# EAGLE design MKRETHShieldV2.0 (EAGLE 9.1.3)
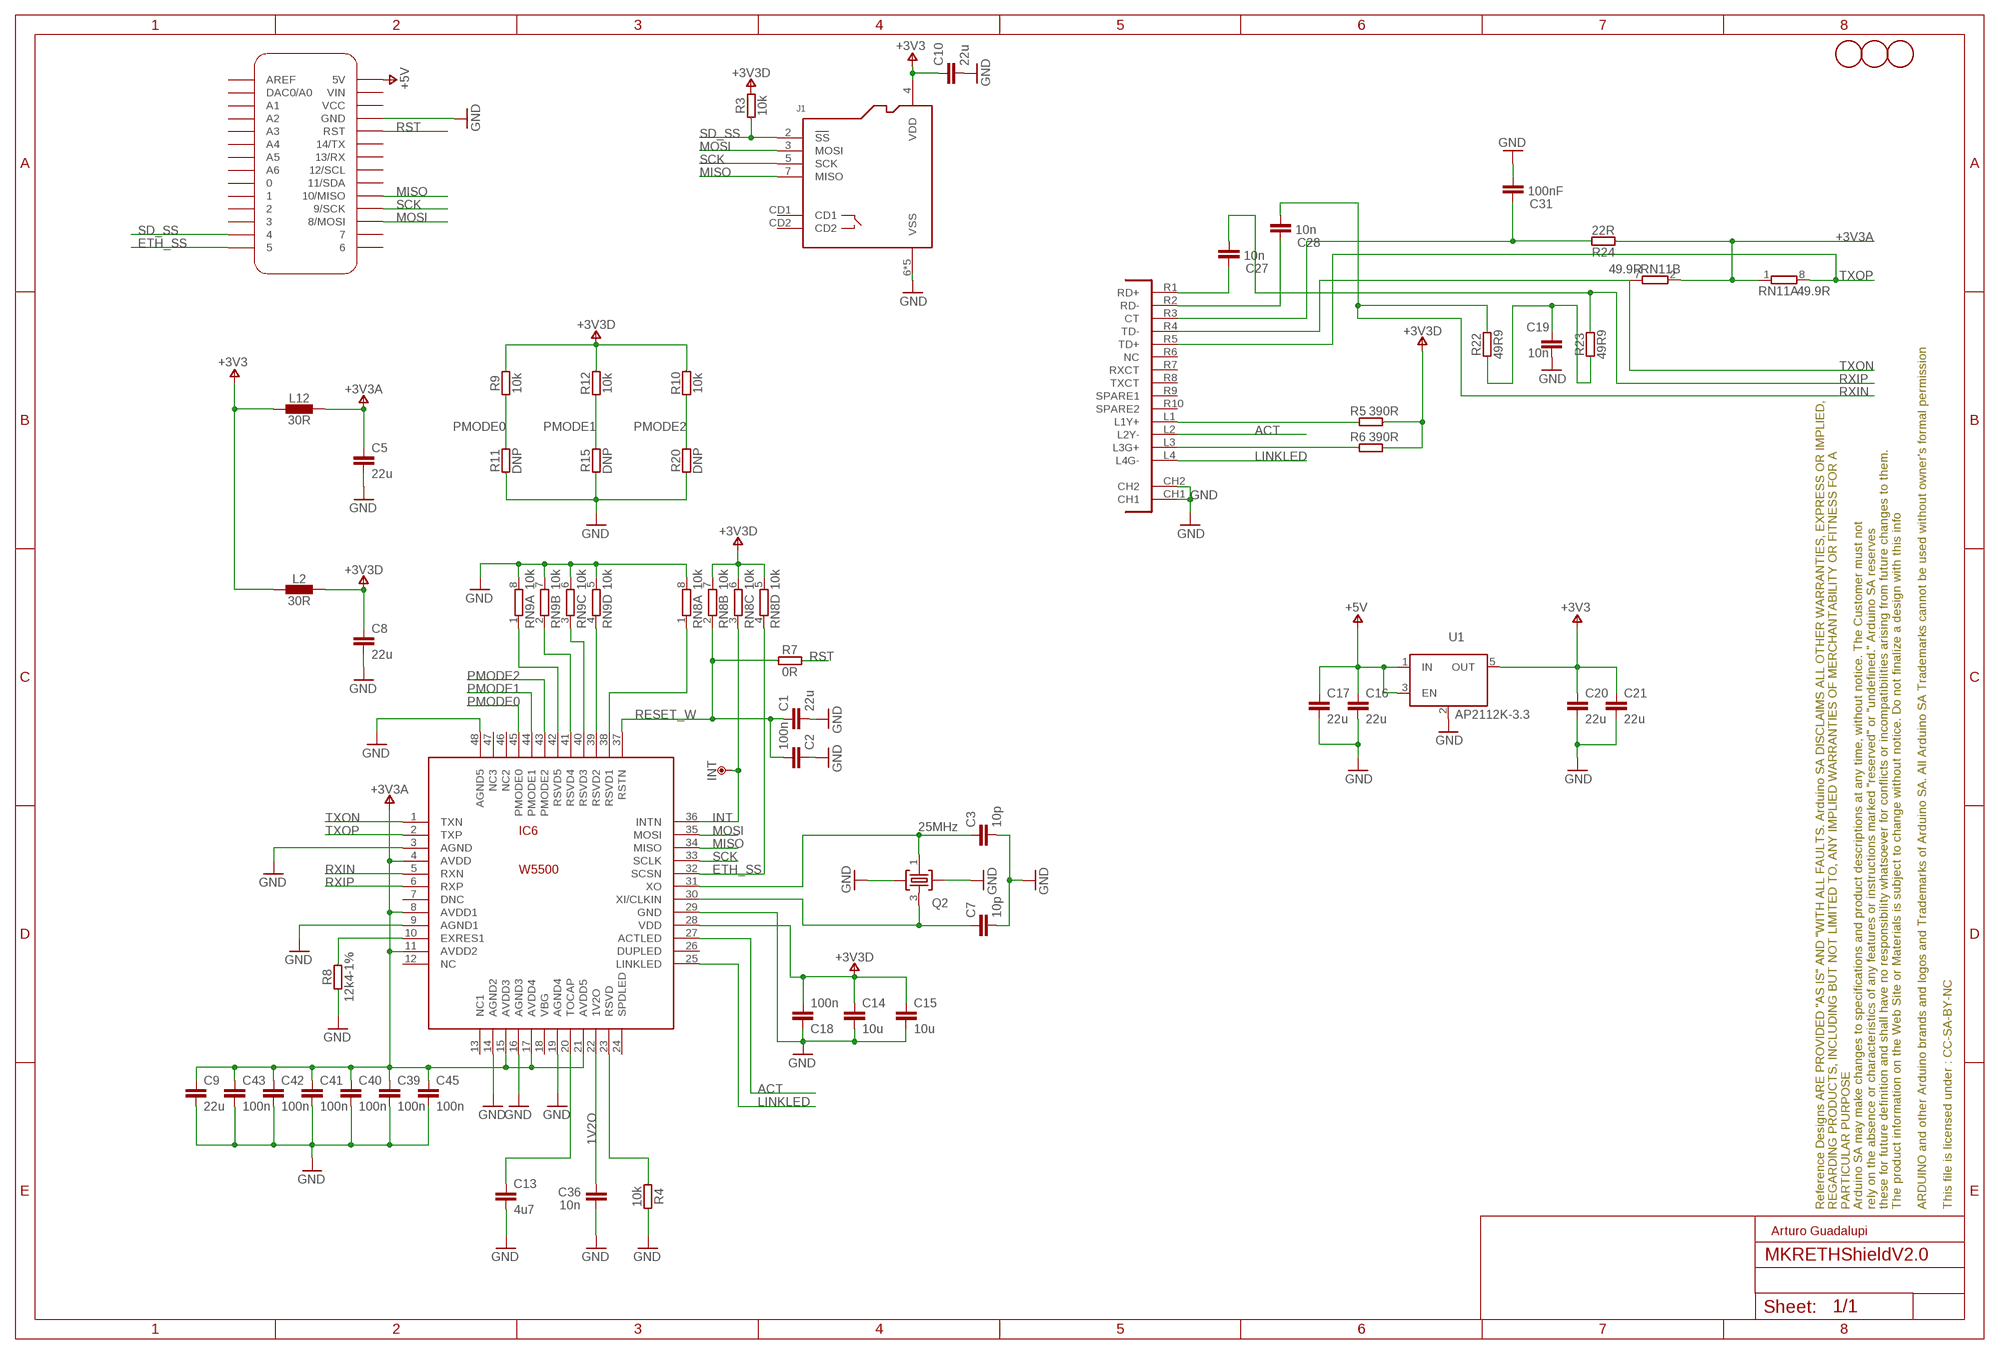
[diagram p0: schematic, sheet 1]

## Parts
C1  22u  C-22U-0805  [0805-R2013X50N]
C2  100n  C-100NF-0402  [0402-1005X55N]
C3  10p  C-10PF-0402  [0402-1005X55N]
C5  22u  C-22U-0805  [0805-R2013X50N]
C7  10p  C-10PF-0402  [0402-1005X55N]
C8  22u  C-22U-0805  [0805-R2013X50N]
C9  22u  C-22U-0805  [0805-R2013X50N]
C10  22u  C-22U-0805  [0805-R2013X50N]
C13  4u7  C-4.7UF-0603  [0603-1608X90N]
C14  10u  C-10UF-0603  [0603-1608X90N]
C15  10u  C-10UF-0603  [0603-1608X90N]
C16  22u  C-22U-0805  [0805-R2013X50N]
C17  22u  C-22U-0805  [0805-R2013X50N]
C18  100n  C-100NF-0402  [0402-1005X55N]
C19  10n  C-10NF-0402  [0402-1005X55N]
C20  22u  C-22U-0805  [0805-R2013X50N]
C21  22u  C-22U-0805  [0805-R2013X50N]
C27  10n  C-10NF-0402  [0402-1005X55N]
C28  10n  C-10NF-0402  [0402-1005X55N]
C31  100nF  C-100NF-0402  [0402-1005X55N]
C36  10n  C-10NF-0402  [0402-1005X55N]
C39  100n  C-100NF-0402  [0402-1005X55N]
C40  100n  C-100NF-0402  [0402-1005X55N]
C41  100n  C-100NF-0402  [0402-1005X55N]
C42  100n  C-100NF-0402  [0402-1005X55N]
C43  100n  C-100NF-0402  [0402-1005X55N]
C45  100n  C-100NF-0402  [0402-1005X55N]
FRAME1  DNP  A3-FRAME-STANDARD  [FRAME]
IC6  W5500  [TQFP48-7X7]
INT  DNP  TPTP-1.27MM  [TP-1.27MM]
J1  -  SD_AMPHENOL-SPI  [AMPHENOL_114-00841-68]
L2  30R  FERRITE-30R0805  [0805-R2013X50N]
L12  30R  FERRITE-30R0805  [0805-R2013X50N]
MKR1  DNP  MKRBOARD-DNP-DIM  [MKRBOARD-DIM]
Q2  25MHz  25MHZ  [CRYSTAL3.2X2.5]
R3  10k  R-10K-0402  [0402-1005X55N]
R4  10k  R-10K-0402  [0402-1005X55N]
R5  390R  R-390R-0402  [0402-1005X55N]
R6  390R  R-390R-0402  [0402-1005X55N]
R7  0R  R-0R-0402  [0402-1005X55N]
R8  12k4-1%  R12K4-1%-0402  [0402-1005X55N]
R9  10k  R-10K-0402  [0402-1005X55N]
R10  10k  R-10K-0402  [0402-1005X55N]
R11  DNP  R-DNP-0402  [0402-1005X55N]
R12  10k  R-10K-0402  [0402-1005X55N]
R15  DNP  R-DNP-0402  [0402-1005X55N]
R20  DNP  R-DNP-0402  [0402-1005X55N]
R22  49R9  R-49R9-0402  [0402-1005X55N]
R23  49R9  R-49R9-0402  [0402-1005X55N]
R24  22R  R-22R-0402  [0402-1005X55N]
RN8  10k  4R-N-10KCAY16  [CAY16]
RN9  10k  4R-N-10KCAY16  [CAY16]
RN11  49.9R  4R-N-49.9RCAY16  [CAY16]
U1  AP2112K-3.3  [SOT25]
U$1  DNP  FIDUCIAL-1.5MM  [FD-1-1.5]
U$2  DNP  FIDUCIAL-1.5MM  [FD-1-1.5]
U$3  DNP  FIDUCIAL-1.5MM  [FD-1-1.5]
UC1  -  ETH-CON-RB1-125BHQ1A  [POE-RJ45]

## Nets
1V2O: C36.2 IC6.22(1V2O)
+3V3 [power]: C10.1 C20.1 C21.1 J1.4(VDD) L2.1 L12.1 U1.5(OUT)
+3V3A [power]: C5.1 C9.1 C39.1 C40.1 C41.1 C42.1 C43.1 C45.1 IC6.4(AVDD) IC6.8(AVDD1) IC6.11(AVDD2) IC6.15(AVDD3) IC6.17(AVDD4) IC6.21(AVDD5) L12.2 R24.1 RN11.1 RN11.2
+3V3D: C8.1 C14.1 C15.1 C18.2 IC6.28(VDD) L2.2 R3.2 R5.2 R6.2 R9.2 R10.2 R12.2 RN8.5 RN8.6 RN8.7
+5V [power]: C16.1 C17.1 MKR1.5V U1.1(IN) U1.3(EN)
ACT: IC6.27(ACTLED) UC1.L2(L2Y-)
ETH_SS: IC6.32(SCSN) MKR1.5 RN8.4
GND [power]: C1.2 C2.1 C3.2 C5.2 C7.2 C8.2 C9.2 C10.2 C13.2 C14.2 C15.2 C16.2 C17.2 C18.1 C19.1 C20.2 C21.2 C31.1 C36.1 C39.2 C40.2 C41.2 C42.2 C43.2 C45.2 IC6.3(AGND) IC6.9(AGND1) IC6.14(AGND2) IC6.16(AGND3) IC6.19(AGND4) IC6.29(GND) IC6.48(AGND5) J1.6(VSS) J1.SH1(VSS) J1.SH2(VSS) J1.SH3(VSS) J1.SH4(VSS) MKR1.GND Q2.2 Q2.4 R4.1 R8.1 R11.1 R15.1 R20.1 RN8.8 RN9.5 RN9.6 RN9.7 RN9.8 U1.2(GND/ADJ) UC1.CH1 UC1.CH2
INT: IC6.36(INTN) INT.X RN8.3
LINKLED: IC6.25(LINKLED) UC1.L4(L4G-)
MISO: IC6.34(MISO) J1.7(MISO) MKR1.10(10/MISO)
MOSI: IC6.35(MOSI) J1.3(MOSI) MKR1.8(8/MOSI)
N$9: C3.1 IC6.31(XO) Q2.1
N$13: IC6.39(RSVD2) RN9.4
N$22: R6.1 UC1.L3(L3G+)
N$24: IC6.23(RSVD) R4.2
N$25: R5.1 UC1.L1(L1Y+)
N$26: C19.2 R22.1 R23.1
N$27: C27.2 UC1.R1(RD+)
N$28: C28.2 UC1.R2(RD-)
N$31: IC6.40(RSVD3) RN9.3
N$35: IC6.41(RSVD4) RN9.2
N$36 [power]: C31.2 R24.2 UC1.R3(CT)
N$37: IC6.42(RSVD5) RN9.1
N$38: C13.1 IC6.20(TOCAP)
N$39: IC6.38(RSVD1) RN8.1
N$40: IC6.10(EXRES1) R8.2
OSC2E2: C7.1 IC6.30(XI/CLKIN) Q2.3
PMODE0: IC6.45(PMODE0) R9.1 R11.2
PMODE1: IC6.44(PMODE1) R12.1 R15.2
PMODE2: IC6.43(PMODE2) R10.1 R20.2
RESET_W: C1.1 C2.2 IC6.37(RSTN) R7.1 RN8.2
RST: MKR1.RST R7.2
RXIN: C28.1 IC6.5(RXN) R22.2
RXIP: C27.1 IC6.6(RXP) R23.2
SCK: IC6.33(SCLK) J1.5(SCK) MKR1.9(9/SCK)
SD_SS: J1.2(SS) MKR1.4 R3.1
TXON: IC6.1(TXN) RN11.7 UC1.R4(TD-)
TXOP: IC6.2(TXP) RN11.8 UC1.R5(TD+)
Unconnected: IC6.7(DNC) IC6.13(NC1) IC6.18(VBG) IC6.24(SPDLED) IC6.46(NC2) IC6.47(NC3) J1.CD1 J1.CD2 MKR1.0 MKR1.1 MKR1.2 MKR1.3 MKR1.6 MKR1.7 MKR1.11(11/SDA) MKR1.12(12/SCL) MKR1.13(13/RX) MKR1.14(14/TX) MKR1.A0(DAC0/A0) MKR1.A1 MKR1.A2 MKR1.A3 MKR1.A4 MKR1.A5 MKR1.A6 MKR1.AREF MKR1.VCC MKR1.VIN RN11.3 RN11.4 RN11.5 RN11.6 UC1.R6(NC) UC1.R7(RXCT) UC1.R8(TXCT) UC1.R9(SPARE1) UC1.R10(SPARE2)

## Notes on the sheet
- Arturo Guadalupi

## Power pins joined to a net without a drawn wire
DUPLED: IC6.26(DUPLED)
NC: IC6.12(NC)

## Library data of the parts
C1 C5 C8-C10 C16 C17 C20 C21 = Arduino-rcl:C: SMD Capacitor; CODE-ARDUINO: 2233; DATASHEET: https://media.digikey.com/pdf/Data%20Sheets/Samsung%20PDFs/CL21A226MQCLQNC_character.pdf; DISTRIBUTOR-LINK: https://www.digikey.com/product-detail/en/samsung-electro-mechanics-america-inc/CL21A226MQCLQNC/1276-2412-1-ND/3890498; DISTRIBUTOR-PN: 1276-2412-1-ND; MANUFACTURER: Samsung; MANUFACTURER-PN: CL21A226MQCLQNC
C2 C18 C31 C39-C43 C45 = Arduino-rcl:C: SMD Capacitor; CODE-ARDUINO: 0132; DATASHEET: http://www.tdk.com/pdf/TDKMLCCCapRange.pdf; DISTRIBUTOR-LINK: http://www.digikey.com/product-detail/en/tdk-corporation/C1005X5R1H104K050BB/445-5942-1-ND/2443982; DISTRIBUTOR-PN: 445-5942-1-ND; MANUFACTURER: TDK; MANUFACTURER-PN: C1005X5R1H104K050BB
C3 C7 = Arduino-rcl:C: SMD Capacitor; CODE-ARDUINO: 3382; DATASHEET: http://search.murata.co.jp/Ceramy/image/img/A01X/partnumbering_e_01.pdf; DISTRIBUTOR-LINK: https://www.digikey.com/product-detail/en/murata-electronics-north-america/GRM1555C1H100FA01D/490-6186-1-ND/3845386; DISTRIBUTOR-PN: 490-6186-1-ND; MANUFACTURER: Murata; MANUFACTURER-PN: GRM1555C1H100FA01D
C13 = Arduino-rcl:C: SMD Capacitor; CODE-ARDUINO: 0458; DATASHEET: http://www.murata.com/~/media/webrenewal/support/library/catalog/products/capacitor/mlcc/c02e.pdf; DISTRIBUTOR-LINK: http://www.digikey.com/product-search/en?keywords=490-7203-1-ND; DISTRIBUTOR-PN: 490-7203-1-ND; MANUFACTURER: Murata; MANUFACTURER-PN: GRM188R61E475KE11D
C14 C15 = Arduino-rcl:C: SMD Capacitor; CODE-ARDUINO: 2213; DATASHEET: http://www.murata.com/~/media/webrenewal/support/library/catalog/products/capacitor/mlcc/c02e.pdf; DISTRIBUTOR-LINK: http://www.digikey.com/product-search/en?keywords=490-10728-1-ND; DISTRIBUTOR-PN: 490-10728-1-ND; MANUFACTURER: Murata; MANUFACTURER-PN: GRM188R61C106KAALD
C19 C27 C28 C36 = Arduino-rcl:C: SMD Capacitor; CODE-ARDUINO: 0165; DATASHEET: http://search.murata.co.jp/Ceramy/image/img/A01X/partnumbering_e_01.pdf; DISTRIBUTOR-LINK: http://www.digikey.com/product-detail/en/murata-electronics-north-america/GRM155R71H103KA88J/490-6351-1-ND/3845548; DISTRIBUTOR-PN: 490-6351-1-ND; MANUFACTURER: Murata; MANUFACTURER-PN: GRM155R71H103KA88J
FRAME1 = Arduino-utility:A3-FRAME: Schematic frame; CODE-ARDUINO: DNP; DATASHEET: DNP; DISTRIBUTOR-LINK: DNP; DISTRIBUTOR-PN: DNP; MANUFACTURER: DNP; MANUFACTURER-PN: DNP
IC6 = Arduino-ICs:W5500: W5500 Hardwired TCP/IP Ethernet controller; CODE-ARDUINO: 0982; DATASHEET: http://wizwiki.net/wiki/lib/exe/fetch.php?media=products:w5500:w5500_ds_v106e_141230.pdf; DISTRIBUTOR-LINK: https://www.digikey.com/product-detail/en/wiznet/W5500/1278-1021-ND/4425702; DISTRIBUTOR-PN: 1278-1021-ND; MANUFACTURER: WizNet; MANUFACTURER-PN: W5500
INT = Arduino-utility:TP: Testpoint; DATASHEET: DNP; DISTRIBUTOR-LINK: DNP; DISTRIBUTOR-PN: DNP; MANUFACTURER: DNP; MANUFACTURER-PN: DNP
J1 = Arduino-connectors:SD_AMPHENOL-SPI: Micro SD connector; CODE-ARDUINO: 0046; DATASHEET: https://www.amphenolcanada.com/ProductSearch/drawings/AC/1140084168.pdf; DISTRIBUTOR-LINK: http://www.digikey.com/product-detail/en/amphenol-commercial-products/114-00841-68/114-00841-68-1-ND/2187101; DISTRIBUTOR-PN: 114-00841-68-1-ND; MANUFACTURER: Amphenol; MANUFACTURER-PN: 114-00841-68
L2 L12 = Arduino-rcl:FERRITE: SMD ferrite; CODE-ARDUINO: 0001; DATASHEET: https://media.digikey.com/pdf/Data%20Sheets/Samsung%20PDFs/Chip_Inductor_Catalog_2014.pdf; DISTRIBUTOR-LINK: https://www.digikey.com/products/en?keywords=CIB21P300NE; DISTRIBUTOR-PN: CIB21P300NE-ND; MANUFACTURER: Samsung; MANUFACTURER-PN: CIB21P300NE
MKR1 = Arduino-utility:MKRBOARD: MKR board footprint; DATASHEET: DNP; DISTRIBUTOR-LINK: DNP; DISTRIBUTOR-PN: DNP; MANUFACTURER: DNP; MANUFACTURER-PN: DNP
Q2 = Arduino-crystals:25MHZ: 25Mhz - K7 12pF - SMD; CODE-ARDUINO: 2359; DATASHEET: https://abracon.com/Resonators/ABM8G.pdf; DISTRIBUTOR-LINK: https://www.digikey.com/product-detail/en/abracon-llc/ABM8G-25.000MHZ-B4Y-T/535-10297-1-ND/2218110; DISTRIBUTOR-PN: 535-10297-1-ND; MANUFACTURER: Abracon LLC; MANUFACTURER-PN: ABM8G-25.000MHZ-B4Y-T
R3 R4 R9 R10 R12 = Arduino-rcl:R: SMD Resistor; CODE-ARDUINO: 0136; DATASHEET: www.yageo.com.tw/exep/pages/download/literatures/PYu-R_INT-thick_7.pdf; DISTRIBUTOR-LINK: http://www.digikey.com/product-detail/en/yageo/RC0402FR-0710KL/311-10.0KLRCT-ND/729470; DISTRIBUTOR-PN: 311-10.0KLRCT-ND; MANUFACTURER: Yageo; MANUFACTURER-PN: RC0402FR-0710KL; _RESTRICTIONS: NO
R5 R6 = Arduino-rcl:R: SMD Resistor; CODE-ARDUINO: 2195; DATASHEET: www.yageo.com.tw/exep/pages/download/literatures/PYu-R_INT-thick_7.pdf; DISTRIBUTOR-LINK: https://www.digikey.com/product-detail/en/yageo/RC0402FR-07390RL/311-390LRCT-ND/2827929; DISTRIBUTOR-PN: 311-390LRCT-ND; MANUFACTURER: Yageo; MANUFACTURER-PN: RC0402FR-07390RL; _RESTRICTIONS: NO
R7 = Arduino-rcl:R: SMD Resistor; CODE-ARDUINO: 0039; DATASHEET: www.yageo.com.tw/exep/pages/download/literatures/PYu-R_INT-thick_7.pdf; DISTRIBUTOR-LINK: http://www.digikey.com/product-detail/en/yageo/RC0402FR-070RL/311-0.0LRCT-ND/2827888; DISTRIBUTOR-PN: 311-0.0LRCT-ND; MANUFACTURER: Yageo; MANUFACTURER-PN: RC0402FR-070RL; _RESTRICTIONS: NO
R8 = Arduino-rcl:R: SMD Resistor; CODE-ARDUINO: 2297; DATASHEET: http://www.yageo.com/NewPortal/yageodocoutput?fileName=/pdf/R-Chip/PYu-RC_Group_51_RoHS_L_4.pdf; DISTRIBUTOR-LINK: https://www.digikey.com/product-detail/en/yageo/RC0402FR-0712K4L/311-12.4KLRCT-ND/2827940; DISTRIBUTOR-PN: 311-12.4KLRCT-ND; MANUFACTURER: Yageo; MANUFACTURER-PN: RC0402FR-0712K4L; _RESTRICTIONS: 1% only
R11 R15 R20 = Arduino-rcl:R: SMD Resistor; CODE-ARDUINO: DNP; DATASHEET: DNP; DISTRIBUTOR-LINK: DNP; DISTRIBUTOR-PN: DNP; MANUFACTURER: DNP; MANUFACTURER-PN: DNP; _RESTRICTIONS: NO
R22 R23 = Arduino-rcl:R: SMD Resistor; CODE-ARDUINO: A5282; DATASHEET: www.yageo.com.tw/exep/pages/download/literatures/PYu-R_INT-thick_7.pdf; DISTRIBUTOR-LINK: https://www.digikey.com/product-detail/en/yageo/RC0402FR-0749R9L/311-49.9LRCT-ND/729568; DISTRIBUTOR-PN: 311-49.9LRCT-ND; MANUFACTURER: Yageo; MANUFACTURER-PN: RC0402FR-0749R9L; _RESTRICTIONS: 1% ONLY
R24 = Arduino-rcl:R: SMD Resistor; CODE-ARDUINO: 0468; DATASHEET: www.yageo.com.tw/exep/pages/download/literatures/PYu-R_INT-thick_7.pdf; DISTRIBUTOR-LINK: http://www.digikey.com/products/en?keywords=311-22.0LRCT-ND; DISTRIBUTOR-PN: 311-22.0LRCT-ND; MANUFACTURER: Yageo; MANUFACTURER-PN: RC0402FR-0722RL; _RESTRICTIONS: NO
RN8 RN9 = Arduino-rcl:4R-N: Array Chip Resistor Source: RS Component / Phycomp; CODE-ARDUINO: 0016; DATASHEET: http://www.bourns.com/docs/Product-Datasheets/CATCAY.pdf; DISTRIBUTOR-LINK: https://www.digikey.com/products/en?keywords=CAY16-103J4LFTR-ND; DISTRIBUTOR-PN: CAY16-103J4LFTR-ND; MANUFACTURER: Bourns Inc.; MANUFACTURER-PN: CAY16-103J4LF
RN11 = Arduino-rcl:4R-N: Array Chip Resistor Source: RS Component / Phycomp; CODE-ARDUINO: 2298; DATASHEET: http://www.bourns.com/docs/Product-Datasheets/CATCAY.pdf; DISTRIBUTOR-LINK: https://www.digikey.com/product-detail/en/bourns-inc/CAY16-49R9F4LF/CAY16-49R9F4LFCT-ND/3437972; DISTRIBUTOR-PN: CAY16-49R9F4LFCT-ND; MANUFACTURER: Bourns Inc.; MANUFACTURER-PN: CAY16-49R9F4LF
U1 = Arduino-ICs:AP2112K-3.3: IC REG LINEAR 3.3V 600mA SOT25; CODE-ARDUINO: 2199; DATASHEET: https://www.diodes.com/assets/Datasheets/AP2112.pdf; DISTRIBUTOR-LINK: https://www.digikey.com/product-detail/en/diodes-incorporated/AP2112K-3.3TRG1/AP2112K-3.3TRG1DITR-ND/4470746; DISTRIBUTOR-PN: AP2112K-3.3TRG1DITR-ND; MANUFACTURER: Diodes Inc; MANUFACTURER-PN: AP2112K-3.3TRG1
U$1-U$3 = Arduino-utility:FIDUCIAL: Fiducial mount; CODE-ARDUINO: DNP; DATASHEET: DNP; DISTRIBUTOR-LINK: DNP; DISTRIBUTOR-PN: DNP; MANUFACTURER: DNP; MANUFACTURER-PN: DNP
UC1 = Arduino-connectors:ETH-CON-RB1-125BHQ1A: RJ45 connector; CODE-ARDUINO: 2300; DATASHEET: https://www2.mouser.com/datasheet/2/443/RB1-125BAG1A(111-00)-1211926.pdf; DISTRIBUTOR-LINK: https://www2.mouser.com/ProductDetail/WIZnet/RB1-125BAG1A?qs=K8aI8m0%252bj2HL3CgJHC4yWQ%3D%3D; DISTRIBUTOR-PN: 950-RB1-125BAG1A; MANUFACTURER: Wiznet; MANUFACTURER-PN: RB1-125BAG1A

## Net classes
1 power: width 0.254 mm, drill 0.3 mm, clearance 0.203 mm
2 gnd: width 0.254 mm, drill 0.3 mm, clearance 0.254 mm

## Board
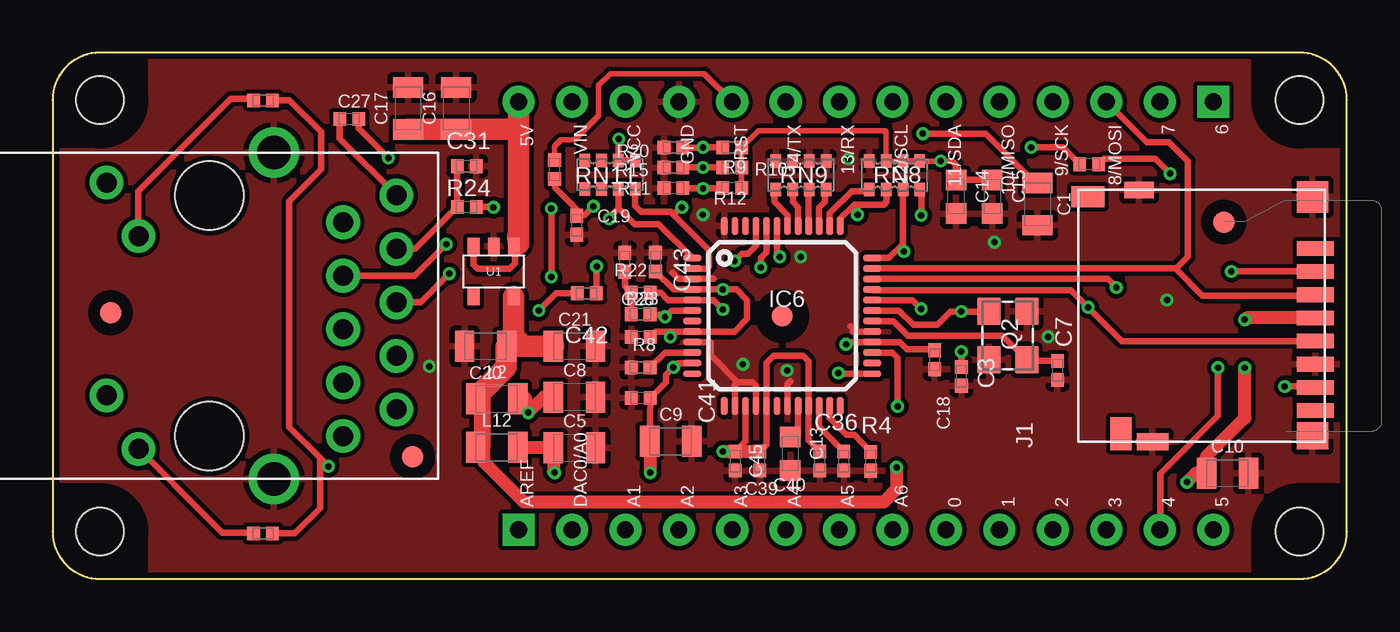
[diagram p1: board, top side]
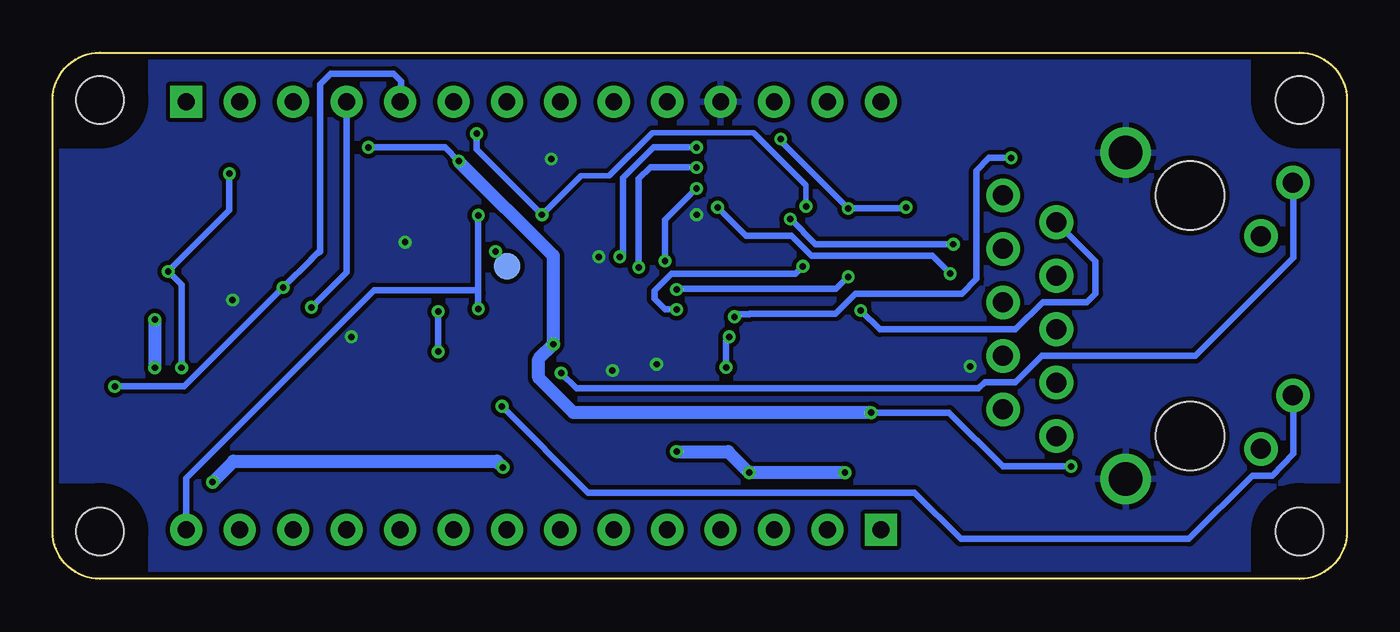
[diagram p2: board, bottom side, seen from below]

Size 61.5 x 25 mm. Coordinates in mm from the lower left corner, seen from the top.
Copper layers (1*16): Top 0.035mm / dielectric 1.5mm / Bottom 0.035mm
Design rules "SeeedStudio_2layers *": minimum track width 6mil, minimum drill 12mil, track to track 7mil, track to pad 6mil, pad to pad 6mil, via to via 6mil, smd to smd 0mil, copper to edge 10mil, drill to drill 10mil, minimum pad ring 10mil, minimum via ring 6mil, stop-mask expansion 2mil, vias tented up to drill 100mil, thermal gap 10mil

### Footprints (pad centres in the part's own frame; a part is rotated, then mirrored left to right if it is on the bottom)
0805-R2013X50N = smd 0.95 x 1.45: 1 -1,0; 2 1,0
0402-1005X55N = smd 0.62 x 0.62: 1 -0.45,0; 2 0.45,0
0603-1608X90N = smd 0.95 x 1: 1 -0.8,0; 2 0.8,0
TQFP48-7X7 = smd 0.85 x 0.32: 1 -4.275,2.75; 2 -4.275,2.25; 3 -4.275,1.75; 4 -4.275,1.25; 5 -4.275,0.75; 6 -4.275,0.25; 7 -4.275,-0.25; 8 -4.275,-0.75; 9 -4.275,-1.25; 10 -4.275,-1.75; 11 -4.275,-2.25; 12 -4.275,-2.75; 25 4.275,-2.75; 26 4.275,-2.25; 27 4.275,-1.75; 28 4.275,-1.25; 29 4.275,-0.75; 30 4.275,-0.25; 31 4.275,0.25; 32 4.275,0.75; 33 4.275,1.25; 34 4.275,1.75; 35 4.275,2.25; 36 4.275,2.75 | smd 0.32 x 0.85: 13 -2.75,-4.275; 14 -2.25,-4.275; 15 -1.75,-4.275; 16 -1.25,-4.275; 17 -0.75,-4.275; 18 -0.25,-4.275; 19 0.25,-4.275; 20 0.75,-4.275; 21 1.25,-4.275; 22 1.75,-4.275; 23 2.25,-4.275; 24 2.75,-4.275; 37 2.75,4.275; 38 2.25,4.275; 39 1.75,4.275; 40 1.25,4.275; 41 0.75,4.275; 42 0.25,4.275; 43 -0.25,4.275; 44 -0.75,4.275; 45 -1.25,4.275; 46 -1.75,4.275; 47 -2.25,4.275; 48 -2.75,4.275 | smd 1 x 1: P$1 0,0
TP-1.27MM = smd 1.27 x 1.27 bottom: X 0,0
AMPHENOL_114-00841-68 = smd 0.7 x 1.75: 1 3.2,-5.888; 2 2.1,-5.888; 3 1,-5.888; 4 -0.1,-5.888; 5 -1.2,-5.888; 6 -2.3,-5.888; 7 -3.4,-5.888; 8 -4.5,-5.888 | smd 1 x 1.55: CD1 5.65,4.912 | smd 1.55 x 1: CD2 -5.602,3.337 | smd 1.3 x 1.5: SH1 -5.7,-5.76 | smd 1.5 x 1.5: SH2 5.65,-5.76 | smd 0.8 x 1.4: SH3 5.975,2.487 | smd 0.8 x 1.5: SH4 -5.975,1.837
MKRBOARD-DIM = drill 0.8 pad 1.524: 0 42.455,2.34; 1 44.995,2.34; 2 47.535,2.34; 3 50.075,2.34; 4 52.615,2.34; 5 55.155,2.34; 5V 22.135,22.66; 7 52.615,22.66; 8 50.075,22.66; 9 47.535,22.66; 10 44.995,22.66; 11 42.455,22.66; 12 39.915,22.66; 13 37.375,22.66; 14 34.835,22.66; A0 24.675,2.34; A1 27.215,2.34; A2 29.755,2.34; A3 32.295,2.34; A4 34.835,2.34; A5 37.375,2.34; A6 39.915,2.34; GND 29.755,22.66; RST 32.295,22.66; VCC 27.215,22.66; VIN 24.675,22.66 | drill 0.8 pad 1.524 square: 6 55.155,22.66; AREF 22.135,2.34 | hole 2.25: 59.25,2.25; 59.25,22.75; 2.25,2.25; 2.25,22.75
CRYSTAL3.2X2.5 = smd 1.3 x 1.1: 1 -1.15,-0.9; 2 1.15,-0.9; 3 1.15,0.9; 4 -1.15,0.9
CAY16 = smd 0.5 x 0.65: 1 -1.2,-0.675; 2 -0.4,-0.675; 3 0.4,-0.675; 4 1.2,-0.675; 5 1.2,0.675; 6 0.4,0.675; 7 -0.4,0.675; 8 -1.2,0.675
SOT25 = smd 0.55 x 0.8: 1 0.95,1.2; 2 0,1.2; 3 -0.95,1.2; 4 -0.95,-1.2; 5 0.95,-1.2
FD-1-1.5 = smd 1.016 x 1.016: P$1 0,0
POE-RJ45 = drill 1.6: CH1 13.94,7.75; CH2 13.94,-7.75 | drill 0.95 pad 1.6: L1 7.51,-6.325; L2 5.99,-3.785; L3 7.51,3.785; L4 5.99,6.325; R1 19.77,5.715; R2 17.23,4.445; R3 19.77,3.175; R4 17.23,1.905; R5 19.77,0.635; R6 17.23,-0.635; R7 19.77,-1.905; R8 17.23,-3.175; R9 19.77,-4.445; R10 17.23,-5.715 | hole 3.25: 10.89,5.715; 10.89,-5.715

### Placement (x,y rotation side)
C1  46.8,17.8 270 top
C2  24.9,16.8 90 top
C3  43.18,9.62 270 top
C5  24.8,6.22 0 top
C7  47.75,9.91 270 top
C8  24.8,8.64 0 top
C9  29.37,6.54 0 top
C10  55.82,5.02 0 top
C13  35.05,5.95 270 top
C14  42.93,18.15 270 top
C15  44.65,18.15 270 top
C16  19.18,22.35 90 top
C17  16.89,22.35 90 top
C18  41.91,10.41 90 top
C19  27.19,15.04 270 top
C20  20.57,11.05 180 top
C21  24.8,11.05 0 top
C27  14.1,21.84 180 top
C28  25.38,13.57 180 top
C31  19.68,19.6 180 top
C36  37.59,5.6 90 top
C39  33.6,5.6 270 top
C40  36.45,5.6 270 top
C41  27.95,8.6 180 top
C42  27.95,11.5 180 top
C43  28.65,15.05 90 top
C45  32.43,5.6 270 top
FRAME1  not placed on the board
IC6  34.67,12.5 0 top
INT  39.9,14.85 0 top
J1  54.1,12.5 90 top
L2  21.1,8.55 0 top
L12  21.1,6.25 0 top
MKR1  0,0 0 top
Q2  45.39,11.56 270 top
R3  49.25,19.7 180 top
R4  38.87,5.59 90 top
R5  10,2.16 0 top
R6  10,22.73 0 top
R7  23.85,19.45 90 top
R8  27.94,10.04 0 top
R9  32.29,18.57 0 top
R10  32.29,20.49 0 top
R11  29.5,18.57 0 top
R12  32.29,19.54 0 top
R15  29.5,19.54 0 top
R20  29.5,20.49 0 top
R22  27.95,13.59 0 top
R23  27.94,12.57 0 top
R24  19.68,17.67 180 top
RN8  40.01,19.18 0 top
RN9  35.56,19.18 0 top
RN11  26.48,19.2 180 top
U1  20.95,14.61 0 top
U$1  2.75,12.65 0 top
U$2  55.65,16.95 0 top
U$3  17.1,5.8 0 top
UC1  -3.43,12.5 0 top

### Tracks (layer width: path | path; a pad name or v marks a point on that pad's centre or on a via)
1V2O
  Top 0.305: IC6.22 36.42,7.22 C36.2
+3V3  (via drill 0.3)
  Top 0.406: 20.5,6.2 20.1,6.2 L12.1 | 20.52,9.02 20.1,9.02 L2.1 | 20.4,8.64 20.1,8.64
  Top 0.61: J1.4 56.72,12.4 v56.64,12.32 | 20.5,6.2 20.5,5.55 22.4,3.65 39.5,3.65 40.1,4.25 v40.1,5.3 | v56.64,10.03 v56.65,10.03 56.65,7.65 54.82,5.82 C10.1 54.32,5.02 v53.9,4.6
  Top 0.813: L12.1 20.4,6.25 20.4,8.64 | 20.1,8.64 L2.1
  Top 1.016: 22.61,11.05 C20.1 21.55,11.03 21.55,10.05 20.52,9.02 | 22.61,11.05 C21.1 | 22.61,11.05 22.34,11.07 21.91,11.5 U1.5
  Bottom 0.61: v56.64,12.32 v56.64,10.03 | v53.9,4.6 52.9,5.6 40.4,5.6 v40.1,5.3
+3V3A  (via drill 0.3)
  Top 0.305: 29.35,11.75 IC6.8 32.4,11.75 33,12.35 33,13.25 32.5,13.75 v31.85,13.75 IC6.4 29.5,13.75 C43.1 | 29.35,11.75 28.65,11.75 C42.1 | RN11.1 RN11.2 26.88,20.88 v26.9,20.9 | C9.1 C41.1 29.15,9.35 29.15,9.7 v29.5,10.05 29.7,10.25 IC6.11 | C39.1 33.92,6.37 IC6.17 33.92,10.27 34.25,10.6 35.65,10.6 35.92,10.33 IC6.21 35.92,6.58 C40.1 | IC6.15 32.92,6.54 C45.1 | R24.1 20.93,17.67 v20.95,17.65 | v29.35,11.5 29.35,11.75 | v23.7,14.35 v23.7,17.6
  Top 0.61: v23.85,5.05 23.8,5.1 C5.1 23.8,6.25 L12.2 | v28.4,5.05 28.4,6.5 C9.1 | v31.85,6.05 C45.1 C39.1
  Bottom 0.305: v31.85,13.75 31.82,13.78 24.27,13.78 v23.7,14.35 | v29.5,10.05 29.5,11.3 v29.35,11.5 | v20.95,17.65 21,17.6 v23.7,17.6 26.9,20.8 v26.9,20.9
  Bottom 0.61: v23.85,5.05 v28.4,5.05 29.4,6.05 v31.85,6.05
+3V3D  (via drill 0.3)
  Top 0.254: R9.2 R12.2 R10.2 33.55,21.3 39.55,21.3 39.6,21.25 RN8.7 RN8.6 | 42.76,19.85 v42.2,19.85 RN8.5
  Top 0.305: C18.2 41.85,10.92 40.59,10.92 40.26,11.25 IC6.28 37.8,11.25 v37.7,11.15 | RN8.6 RN8.5 | 42.76,19.85 42.93,19.68 C14.1 C15.1 | v46.5,20.5 48,20.5 R3.2 | R5.2 11.51,2.16 12.7,3.35 12.7,5.75 | 12.7,5.75 11.25,7.2 11.25,17.95 12.75,19.45 12.75,21.25 11.25,22.75 10.47,22.75 R6.2 | 12.7,5.75 v13.1,5.35
  Top 0.406: 22.37,8.55 22.6,8.55 v22.6,7.9
  Top 0.61: C8.1 23.34,8.64 v22.6,7.9
  Top 0.813: L2.2 22.37,8.55
  Bottom 0.305: v46.5,20.5 42.85,20.5 v42.2,19.85 | v22.6,7.9 18.9,7.9 16.35,5.35 v13.1,5.35
  Bottom 0.61: v42.2,19.85 37.7,15.35 v37.7,11.15 38.4,10.45 38.4,9.55 36.75,7.9 v22.6,7.9
+5V
  Top 0.305: 22.14,16.38 21.91,16.15 U1.1 21.97,15.74 21.97,14.99 21.72,14.73 20.19,14.73 20,14.92 U1.3
  Top 1.016: C17.1 C16.1 21.86,21.35 22.14,21.08 | MKR1.5V 22.14,21.08 | 22.14,21.08 22.14,16.38 22.14,15.91 22.1,16.26
ACT  (via drill 0.3)
  Top 0.305: v40.15,8.2 40.15,10.5 39.9,10.75 IC6.27
  Bottom 0.305: v40.15,8.2 36.05,4.1 20.55,4.1 18.35,1.9 7.5,1.9 4.5,4.9 3.55,4.9 2.55,5.95 UC1.L2
ETH_SS  (via drill 0.3)
  Top 0.305: IC6.32 40.85,13.25 v41.27,12.83 | v41.27,17.27 41.27,18.43 RN8.4
  Bottom 0.305: v41.27,12.83 41.27,13.59 | 41.27,13.59 v41.27,17.27 | MKR1.5 55.16,4.79 46.23,13.72 41.4,13.72 41.27,13.59
GND  (via drill 0.3)
  Top 0.305: IC6.19 34.92,9.27 35.05,9.4 | 38.04,11.75 IC6.29 38.15,11.75 37.9,12 | IC6.9 31.25,11.25 31.25,10.65 32.55,9.35 | 31.4,14.25 IC6.3 | IC6.3 30.35,14.25 | IC6.3 29.75,14.25 29.45,14.55 | 32.4,9.1 32.42,9.08 IC6.14 32.42,9.22 32.55,9.35 | 32.55,9.35 33.25,9.35 33.42,9.18 IC6.16
  other vias: 44.75,16 35.55,15.3 30.9,17.3 52.95,13.25 37.8,19.95 34.9,9.9 17.9,10.1 47.3,11.5 32.8,10.2
  pour Top: 0,25 62,25 62,0 0,0
  pour Bottom: 0,25 62,25 62,0 0,0
INT  (via drill 0.3)
  Top 0.305: RN8.3 40.41,15.9 | 40.41,15.9 39.75,15.25 IC6.36 | 40.41,15.9 40.41,15.6 v40.45,15.55
  Bottom 0.305: v40.45,15.55 INT.X
LINKLED  (via drill 0.3)
  Top 0.305: v37.34,9.78 37.37,9.75 IC6.25 39.02,9.75
  Bottom 0.305: v37.34,9.78 36.61,9.05 17.5,9.05 17.2,9.35 15.75,9.35 14.5,10.6 7.2,10.6 2.55,15.25 UC1.L4
MISO  (via drill 0.3)
  Top 0.305: v58.55,9.14 59.95,9.14 J1.7 | IC6.34 50.14,14.25 v50.54,13.85
  Bottom 0.305: v58.55,9.14 55.24,9.14 v50.54,13.85 49.2,15.19 49.2,15.2 48.9,15.5 48.85,15.5 48.8,15.55 48.8,23.5 48.3,24 45.3,24 44.95,23.65 44.95,22.7 MKR1.10
MOSI
  Top 0.305: IC6.35 53.35,14.75 | J1.3 59.95,13.46 54.64,13.46 53.35,14.75 | 50.05,22.64 MKR1.8 51.98,20.75 53.05,20.75 53.95,19.85 53.95,15.3 53.4,14.75 53.35,14.75
N$9  (via drill 0.3)
  Top 0.305: IC6.31 40.21,12.75 40.89,12.06 42.04,12.06 42.67,12.7 v43.18,12.7 44.74,12.7 Q2.1 | C3.1 v43.18,10.79
  Bottom 0.305: v43.18,10.79 v43.18,12.7
N$13
  Top 0.305: IC6.39 36.42,17.62 36.7,17.91 36.7,18.45 RN9.4
N$22
  Top 0.305: UC1.L3 4.06,16.3 4.06,18.41 8.45,22.8 9.48,22.8 R6.1
N$24
  Top 0.305: IC6.23 36.92,7.66 37.72,6.86 38.1,6.86 R4.2
N$25
  Top 0.305: UC1.L1 7.4,2.85 7.66,2.6 8.06,2.2 9.51,2.2 R5.1
N$26
  Top 0.305: 27.44,13.66 R22.1 | R22.1 27.5,12.59 R23.1 | C19.2 27.19,13.9 R22.1
N$27
  Top 0.305: C27.2 13.65,20.91 UC1.R1
N$28  (via drill 0.3)
  Top 0.305: C28.2 23.92,13.57 v23.1,12.75
  Bottom 0.305: UC1.R2 11.95,15.09 11.95,13.55 12.35,13.15 14.45,13.15 15.75,11.85 22.2,11.85 v23.1,12.75
N$31
  Top 0.305: IC6.40 35.92,18.46 RN9.3
N$35
  Top 0.305: IC6.41 35.42,17.66 35.18,17.91 35.18,18.48 RN9.2
N$36
  Top 0.305: UC1.R3 17.23,15.68 R24.2 C31.2
N$37
  Top 0.305: IC6.42 34.92,17.28 34.29,17.91 34.29,18.43 RN9.1
N$38
  Top 0.305: IC6.20 35.42,6.77 C13.1
N$39
  Top 0.305: IC6.38 36.92,17.36 37.97,18.41 38.72,18.41 RN8.1
N$40
  Top 0.305: IC6.10 29.09,10.75 R8.2
OSC2E2
  Top 0.305: IC6.30 39.95,12.25 40.64,11.56 45.14,11.56 Q2.3 46.34,10.36 C7.1
PMODE0  (via drill 0.3)
  Top 0.305: R11.2 30.88,18.57 v30.91,18.55 31.82,18.55 R9.1 | IC6.45 33.42,15.82 33.05,15.45 32.75,15.45 v32.4,15.1
  Bottom 0.305: v32.4,15.1 32.4,17.06 v30.91,18.55
PMODE1  (via drill 0.3)
  Top 0.305: R12.1 v30.91,19.54 R15.2 | IC6.44 33.92,15.52 33.65,15.25 v33.65,14.8
  Bottom 0.305: v33.65,14.8 33.65,19 33.1,19.55 31.36,19.55 31.35,19.54 v30.91,19.54
PMODE2  (via drill 0.3)
  Top 0.305: R20.2 30.8,20.49 v30.91,20.5 R10.1 | IC6.43 34.42,15.43 v34.55,15.3
  Bottom 0.305: v34.55,15.3 34.4,15.45 34.4,19.05 32.95,20.5 v30.91,20.5 30.8,20.49
RESET_W  (via drill 0.3)
  Top 0.254: R7.1 23.85,18.6 24.9,17.55 C2.2 25.25,17.25 v25.7,17.7
  Top 0.305: IC6.37 37.42,17.1 38.1,17.78 38.25,17.78 | 38.25,17.78 39.5,17.78 39.62,17.91 39.62,18.48 RN8.2 | v38.25,17.3 38.25,17.78 | v41.35,21.15 44.35,21.15 46.4,19.1 46.5,19.1 C1.1
  Bottom 0.254: v25.7,17.7 25.7,18.7 28.2,21.2 33,21.2 35.05,19.15 36.4,19.15 v38.25,17.3
  Bottom 0.305: v41.35,21.15 41.35,20.4 v38.25,17.3
RST
  Top 0.254: R7.2 23.85,20.55 24.15,20.85 24.8,20.85 25.95,22 25.95,23.45 26.5,24 30.95,24 MKR1.RST
RXIN  (via drill 0.3)
  Top 0.305: R22.2 28.91,13.59 29.25,13.25 IC6.5 31.4,13.25 v31.85,12.8 | v25.85,14.85 25.85,13.59 C28.1
  Bottom 0.305: v31.85,12.8 32.4,12.8 32.9,13.3 32.9,13.7 32.1,14.5 26.2,14.5 v25.85,14.85
RXIP  (via drill 0.3)
  Top 0.305: C27.1 14.55,21.4 v15.95,20 | R23.2 28.41,12.55 29,12.55 v29.1,12.45 29.4,12.75 IC6.6
  Bottom 0.305: v15.95,20 17,20 17.6,19.4 17.6,14.25 18.3,13.55 23.35,13.55 24.3,12.6 28.36,12.6 R23.2 28.98,12.57 v29.1,12.45
SCK  (via drill 0.3)
  Top 0.305: IC6.33 38.98,13.72 48.38,13.72 v49.2,12.9 50.8,11.3 J1.5
  Bottom 0.305: MKR1.9 47.53,14.56 v49.2,12.9
SD_SS  (via drill 0.3)
  Top 0.254: MKR1.4 52.63,2.34
  Top 0.305: v55.37,10.03 55.37,7.75 52.63,5.01 52.63,2.34 | v56.01,14.61 J1.2 | v53.1,19.25 52.4,19.95 49.95,19.95 R3.1
  Bottom 0.305: v55.37,10.03 55.37,13.97 v56.01,14.61 53.1,17.51 v53.1,19.25
TXON  (via drill 0.3)
  Top 0.305: IC6.1 28.8,16.85 27.65,16.85 26.88,17.62 | RN11.7 26.88,17.62 | UC1.R4 17.2,14.4 v18.7,15.9 | v26.45,17.1 26.45,17.18 26.88,17.62
  Bottom 0.305: v18.7,15.9 25.25,15.9 v26.45,17.1
TXOP  (via drill 0.3)
  Top 0.305: 29.51,17.31 29.36,17.45 27.95,17.45 27.68,17.72 RN11.8 | 29.51,17.31 31.19,15.62 31.19,14.86 31.07,14.73 30.41,14.73 IC6.2 | UC1.R5 17.48,13.13 v18.85,14.5 | v29.9,17.65 29.85,17.65 29.51,17.31
  Bottom 0.305: v29.9,17.65 28.55,16.3 26.4,16.3 25.45,15.35 19.7,15.35 v18.85,14.5

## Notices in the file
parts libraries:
Arduino-rcl: Copyright (c) 2016-2017 Arduino LLC. All right reserved.
Arduino-utility: This file is licensed under : CC-SA-BY-NC
